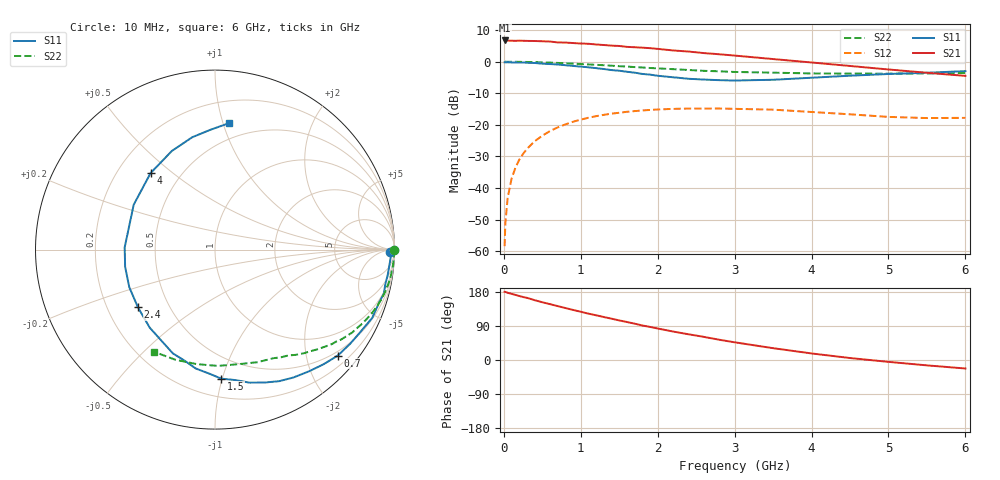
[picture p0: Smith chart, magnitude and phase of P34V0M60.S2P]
! SIEMENS Small Signal Semiconductors
! BFP181
! Si NPN RF Bipolar Junction Transistor in SOT143
! VCE = 4 V  IC = 0.6 mA
! Common Emitter S-Parameters:  March  1996
# GHz  S  MA  R  50
!  f  S11  S21  S12  S22
! GHz  MAG  ANG  MAG  ANG  MAG  ANG  MAG  ANG
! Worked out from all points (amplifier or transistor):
!   36 points, 10 MHz to 6 GHz, reference 50 ohm
!   highest |S21| = 6.7 dB at 10 MHz (marker M1)
!   |S21| within 3 dB of that: start of sweep to 2.135 GHz
!   unconditionally stable (mu >= 1): 3.658 GHz to end of sweep
!   at 250 MHz: K = 0.08, MSG = 17.9 dB, |S12| = -29.2 dB
!   at 1.4 GHz: K = 0.44, MSG = 10.8 dB, |S12| = -16.4 dB
!   at 6 GHz: K = 1.38, MAG = 3.0 dB, |S12| = -17.8 dB
!   S11 on the Smith chart (normalised r, x): 10 MHz: 64, -40; 700 MHz: 0.41, -2.63; 1.5 GHz: 0.33, -0.99; 2.4 GHz: 0.33, -0.30; 4 GHz: 0.34, +0.42; 6 GHz: 0.37, +1.05
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0.01  0.9777 -0.8  2.169 179.8  0.0012 79.8  0.999 -0.2
0.02  0.9764 -1.2  2.147 179.7  0.0028 87.3  0.9986 -0.6
0.05  0.9794 -2.8  2.156 177.4  0.007 91.2  0.9978 -1.4
0.1  0.9746 -6.0  2.15 174.5  0.014 84.4  0.9972 -2.8
0.15  0.9722 -8.7  2.139 171.9  0.0208 83.4  0.996 -4.2
0.25  0.9723 -14.6  2.145 166.2  0.0347 79.9  0.9917 -7.1
0.4  0.9549 -23.5  2.126 157.9  0.055 74.1  0.9847 -11.2
0.6  0.9176 -35.0  2.085 147.4  0.0797 65.6  0.9677 -16.6
0.7  0.9037 -40.8  2.02 142.2  0.0911 61.7  0.9564 -19.3
0.9  0.857 -52.3  1.974 132.1  0.1121 54.0  0.9326 -24.0
1.1  0.8156 -64.0  1.921 122.3  0.1297 46.9  0.9051 -28.8
1.5  0.7198 -87.2  1.774 104.4  0.1555 34.2  0.8483 -37.1
1.9  0.6244 -112.0  1.639 87.3  0.1722 23.2  0.7952 -44.4
2.2  0.5669 -129.9  1.507 75.1  0.179 16.4  0.7611 -49.3
2.4  0.5364 -143.2  1.448 67.9  0.1809 11.8  0.7392 -52.5
2.8  0.5099 -169.1  1.312 53.5  0.1814 4.3  0.7043 -58.4
3  0.5034 178.6  1.25 46.7  0.1793 0.5  0.688 -61.5
3.5  0.5174 151.1  1.101 31.2  0.174 -6.5  0.6707 -69.3
4  0.5573 130.1  0.972 17.3  0.1599 -11.5  0.6515 -78.5
4.5  0.6 113.6  0.856 5.2  0.1469 -14.9  0.6482 -88.6
5.5  0.6685 92.1  0.668 -14.2  0.1281 -10.9  0.6523 -109.8
6  0.709 83.6  0.596 -22.4  0.1291 -7.4  0.6631 -120.9
